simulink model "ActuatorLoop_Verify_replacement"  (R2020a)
settings: Solver=FixedStepDiscrete  StartTime=0.0  StopTime=10.0  FixedStep=0.001  RelTol=1e-3
model workspace (MAT data in the model file):
  Kd : Simulink.Parameter (value not decoded)
  Ki : Simulink.Parameter (value not decoded)
  Kp : Simulink.Parameter (value not decoded)
  Ts : Simulink.Parameter (value not decoded)
symbols that are objects in the model workspace (value not decoded): Kd, Ki, Kp, Ts
undefined symbols (not defined in the file or in its folder): ActuatorLoop, ActuatorLoop_New, ActuatorLoop_Original, DiscIntNeverNeededParam, Normal, sldvsubsys
libraries: simulink x4, sldvlib x1

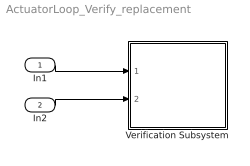
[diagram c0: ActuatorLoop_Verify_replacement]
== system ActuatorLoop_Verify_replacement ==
  In1 : Inport
  In2 : Inport  Port=2
  Verification Subsystem : Subsystem  Tag=VerificationSubsystem  DisableCoverage=on  LoadFcn=sldvsubsys('check')  TreatAsAtomicUnit=on  SimViewingDevice=on  mask(VerificationSubsystem){}
      mask init:
      | sldvsubsys('maskInit');
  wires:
  In1/1 -> Verification Subsystem/1(In1)
  In2/1 -> Verification Subsystem/2(In2)

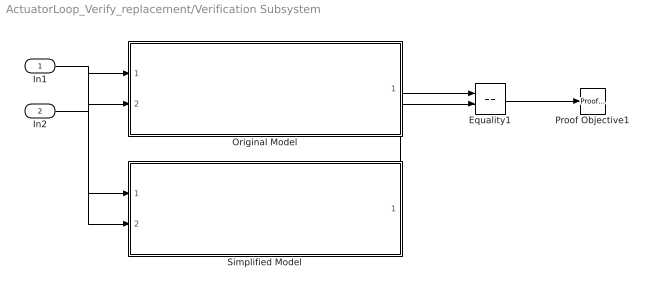
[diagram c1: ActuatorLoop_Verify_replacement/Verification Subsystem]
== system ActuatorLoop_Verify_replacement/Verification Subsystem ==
  In1 : Inport
  In2 : Inport  Port=2
  Equality1 : RelationalOperator  Operator===  OutDataTypeStr=boolean  RndMeth=Simplest
  Original Model : Subsystem  TreatAsAtomicUnit=on  mask(Sldv ModelReference(Model name:ActuatorLoop_Original) Replacement){ModelName=ActuatorLoop_Original, ParameterArgumentNames=, ParameterArgumentValuesAsString=, SimulationMode=Normal}
      mask help: Replacement for the Model Reference block that references the model ActuatorLoop_Original. If Model arguments are specified on the Model Reference block, then they will appear in the mask parameters.
  Proof Objective1 : sldvlib/Objectives and Constraints/Proof Objective  enabled=on  customAVTBlockType=Proof Objective  intervals=true  dispValues=on  outEnabled=off  enableStopSim=off
  Simplified Model : Subsystem  TreatAsAtomicUnit=on  mask(Sldv ModelReference(Model name:ActuatorLoop_New) Replacement){ModelName=ActuatorLoop_New, ParameterArgumentNames=, ParameterArgumentValuesAsString=, SimulationMode=Normal}
      mask help: Replacement for the Model Reference block that references the model ActuatorLoop_New. If Model arguments are specified on the Model Reference block, then they will appear in the mask parameters.
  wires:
  In1/1 -> Original Model/1(PositionFeedback), Simplified Model/1(PositionFeedback)
  In2/1 -> Original Model/2(PositionCommand), Simplified Model/2(PositionCommand)
  Original Model/1(ActuatorCommand) -> Equality1/1
  Simplified Model/1(ActuatorCommand) -> Equality1/2
  Equality1/1 -> Proof Objective1/1

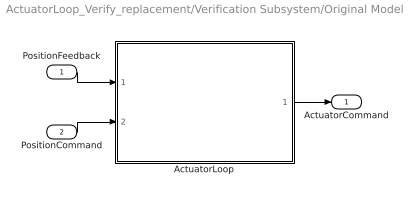
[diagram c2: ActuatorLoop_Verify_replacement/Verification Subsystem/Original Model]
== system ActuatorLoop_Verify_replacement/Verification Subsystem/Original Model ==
  PositionFeedback : Inport  OutMin=-32768  OutMax=32767  OutDataTypeStr=int16  PortDimensions=1  SampleTime=[0.001,0]
  PositionCommand : Inport  Port=2  OutMin=-0.1  OutMax=0.1  OutDataTypeStr=double  PortDimensions=1  SampleTime=[0.001,0]
  ActuatorLoop : Subsystem  TreatAsAtomicUnit=on  mask(Sldv ModelReference(Model name:ActuatorLoop) Replacement){Kd=double(0.00272), Ki=double(2.73), Kp=double(0.339), ModelName=ActuatorLoop, ParameterArgumentNames=Kd,Ki,Kp, ParameterArgumentValuesAsString=0.00272,2.73,0.339, SimulationMode=Normal}
      mask help: Replacement for the Model Reference block that references the model ActuatorLoop. If Model arguments are specified on the Model Reference block, then they will appear in the mask parameters.
  ActuatorCommand : Outport  OutDataTypeStr=int16  PortDimensions=1  SampleTime=[0.001,0]  VectorParamsAs1DForOutWhenUnconnected=off
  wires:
  ActuatorLoop/1(ActuatorCommand) -> ActuatorCommand/1
  PositionFeedback/1 -> ActuatorLoop/1(PositionFeedback)
  PositionCommand/1 -> ActuatorLoop/2(PositionCommand)

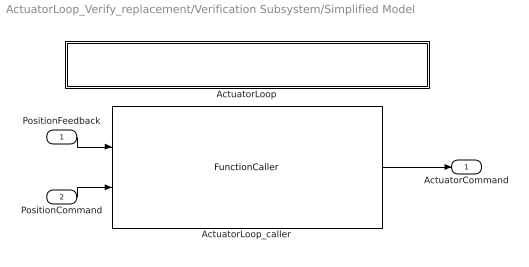
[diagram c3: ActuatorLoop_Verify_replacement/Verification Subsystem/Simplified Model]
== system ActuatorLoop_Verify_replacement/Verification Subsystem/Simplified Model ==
  PositionFeedback : Inport  OutMin=-32768  OutMax=32767  OutDataTypeStr=int16  PortDimensions=1  SampleTime=[0.001,0]
  PositionCommand : Inport  Port=2  OutMin=-0.1  OutMax=0.1  OutDataTypeStr=double  PortDimensions=1  SampleTime=[0.001,0]
  ActuatorLoop : Subsystem  TreatAsAtomicUnit=on
  ActuatorLoop_caller : FunctionCaller  FunctionPrototype=ActuatorCommand = ActuatorLoop(PositionFeedback,PositionCommand)  InputArgumentSpecifications=int16(1), double(1)  OutputArgumentSpecifications=int16(1)
  ActuatorCommand : Outport  OutDataTypeStr=int16  PortDimensions=1  SampleTime=[0.001,0]  VectorParamsAs1DForOutWhenUnconnected=off
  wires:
  ActuatorLoop_caller/1 -> ActuatorCommand/1
  PositionFeedback/1 -> ActuatorLoop_caller/1
  PositionCommand/1 -> ActuatorLoop_caller/2

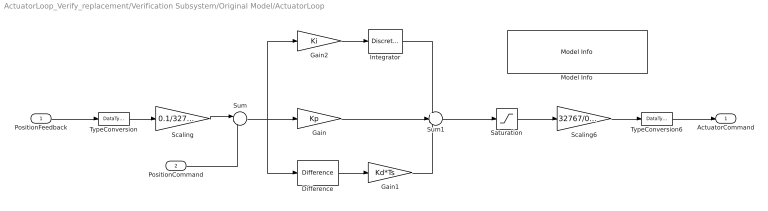
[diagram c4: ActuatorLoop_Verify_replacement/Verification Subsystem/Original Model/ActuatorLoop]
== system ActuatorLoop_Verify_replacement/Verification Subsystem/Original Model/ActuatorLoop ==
  PositionFeedback : Inport  OutMin=-32768  OutMax=32767  OutDataTypeStr=int16  PortDimensions=1  SampleTime=[0.001,0]
  PositionCommand : Inport  Port=2  OutMin=-0.1  OutMax=0.1  OutDataTypeStr=double  PortDimensions=1  SampleTime=[0.001,0]
  Difference : simulink/Discrete/Difference  ICPrevInput=0.0  OutMin=[]  OutMax=[]  OutDataType=fixdt(1, 16)  OutScaling=2^-10  DoSatur=off
  Gain : Gain  Gain=Kp
  Gain1 : Gain  Gain=Kd*Ts
  Gain2 : Gain  Gain=Ki
  Integrator : DiscreteIntegrator  SampleTime=-1  LimitOutput=on  UpperSaturationLimit=0.1  LowerSaturationLimit=-0.1  ICPrevOutput=DiscIntNeverNeededParam  ICPrevScaledInput=DiscIntNeverNeededParam
  Model Info : simulink/Model-Wide Utilities/Model Info  Frame=on  DisplayStringWithTags=|  HorizontalTextAlignment=Center  LeftAlignmentValue=0.5
      | Model Name: %<ModelName>
      | Model Version: %<ModelVersion>
      | Last Modified: %<LastModificationDate>
      | 
      | Copyright 2016 The MathWorks, Inc.
  Saturation : Saturate  UpperLimit=0.3  LowerLimit=-0.3
  Scaling : Gain  Gain=0.1/32767
  Scaling6 : Gain  Gain=32767/0.3  SaturateOnIntegerOverflow=on
  Sum : Sum  Inputs=|-+
  Sum1 : Sum  Inputs=++-
  TypeConversion : DataTypeConversion  OutDataTypeStr=double
  TypeConversion6 : DataTypeConversion  OutDataTypeStr=int16
  ActuatorCommand : Outport  OutDataTypeStr=int16  PortDimensions=1  SampleTime=[0.001,0]  VectorParamsAs1DForOutWhenUnconnected=off
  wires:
  TypeConversion6/1 -> ActuatorCommand/1
  Saturation/1 -> Scaling6/1
  Scaling6/1 -> TypeConversion6/1
  Scaling/1 -> Sum/1
  TypeConversion/1 -> Scaling/1
  PositionFeedback/1 -> TypeConversion/1
  Gain2/1 -> Integrator/1
  Gain1/1 -> Sum1/3
  Difference/1 -> Gain1/1
  Integrator/1 -> Sum1/1
  Sum1/1 -> Saturation/1
  Gain/1 -> Sum1/2
  Sum/1 -> Difference/1, Gain2/1, Gain/1
  PositionCommand/1 -> Sum/2

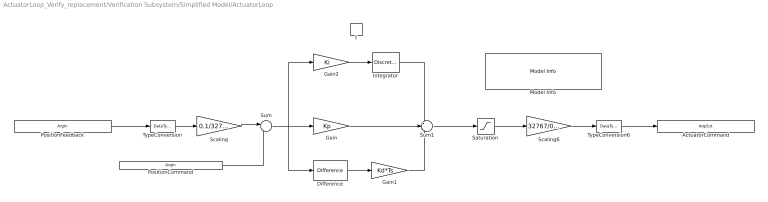
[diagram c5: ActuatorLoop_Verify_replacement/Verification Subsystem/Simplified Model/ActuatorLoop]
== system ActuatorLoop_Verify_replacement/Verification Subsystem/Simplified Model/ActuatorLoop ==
  f : TriggerPort  TriggerType=function-call  IsSimulinkFunction=on  FunctionName=ActuatorLoop  FunctionVisibility=scoped  VariantControl=Variant  PortDimensions=1
  Difference : simulink/Discrete/Difference  ICPrevInput=0.0  OutMin=[]  OutMax=[]  OutDataType=fixdt(1, 16)  OutScaling=2^-10  DoSatur=off
  Gain : Gain  Gain=Kp
  Gain1 : Gain  Gain=Kd*Ts
  Gain2 : Gain  Gain=Ki
  Integrator : DiscreteIntegrator  SampleTime=-1  LimitOutput=on  UpperSaturationLimit=0.1  LowerSaturationLimit=-0.1  ICPrevOutput=DiscIntNeverNeededParam  ICPrevScaledInput=DiscIntNeverNeededParam
  Model Info : simulink/Model-Wide Utilities/Model Info  Frame=on  DisplayStringWithTags=|  HorizontalTextAlignment=Center  LeftAlignmentValue=0.5
      | Model Name: %<ModelName>
      | Model Version: %<ModelVersion>
      | Last Modified: %<LastModificationDate>
      | 
      | Copyright 2016 The MathWorks, Inc.
  Saturation : Saturate  UpperLimit=0.3  LowerLimit=-0.3
  Scaling : Gain  Gain=0.1/32767
  Scaling6 : Gain  Gain=32767/0.3  SaturateOnIntegerOverflow=on
  Sum : Sum  Inputs=|-+
  Sum1 : Sum  Inputs=++-
  TypeConversion : DataTypeConversion  OutDataTypeStr=double
  TypeConversion6 : DataTypeConversion  OutDataTypeStr=int16
  PositionFeedback : ArgIn  OutMin=-32768  OutMax=32767  OutDataTypeStr=int16  ArgumentName=PositionFeedback
  PositionCommand : ArgIn  Port=2  OutMin=-0.1  OutMax=0.1  ArgumentName=PositionCommand
  ActuatorCommand : ArgOut  OutDataTypeStr=int16  ArgumentName=ActuatorCommand
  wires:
  Gain/1 -> Sum1/2
  PositionCommand/1 -> Sum/2
  Gain2/1 -> Integrator/1
  Scaling6/1 -> TypeConversion6/1
  PositionFeedback/1 -> TypeConversion/1
  Gain1/1 -> Sum1/3
  Sum1/1 -> Saturation/1
  Scaling/1 -> Sum/1
  Sum/1 -> Difference/1, Gain2/1, Gain/1
  Integrator/1 -> Sum1/1
  TypeConversion/1 -> Scaling/1
  TypeConversion6/1 -> ActuatorCommand/1
  Difference/1 -> Gain1/1
  Saturation/1 -> Scaling6/1
